| IBIS file generated by GenIBIS.exe Version 2.20
|   am37xxcbc
[IBIS ver]   4.1
[File name]   sprm510.ibs
[File Rev]   1.0
[Date]   Fri Jun 4, 2010, 5:00:00
[Source]   Data created at Texas Instruments
[Notes]   1) IBIS spec conformance checker (IBISCK4) ran with 0 errors
   and 576 warnings.  Warnings should be waived.
[Disclaimer] Please be aware that in the absence of a written agreement,
   Texas Instruments (TI) assumes no liability for: 1) the
   accuracy of the IBIS models provided to your company, 2) the
   proper functioning of these IBIS models in your design or for
   any resulting applications, or, 3) infringement of patents,
   copyrights, or intellectual property rights resulting from
   your use of these IBIS models. TI provides IBIS models as a
   service to our customers and therefore reserves the right to
   limit distribution of the IBIS models.
[Copyright]   Property of Texas Instruments Incorporated. Unauthorised
   reproduction and/or distribution is strictly prohibited. This
   product is protected under copyright law and trade secret law
   as an unpublished work. Created 1999,(C) Copyright 1999-2001,
   Texas Instruments Incorporated., All Rights Reserved. These
   commodities are under the U.S. Government distribution license
   control.As such,they are not to be re-exported without the
   prior approval of the U.S. Department of Commerce.
|   Component am37xxcbc
[Component]   am37xxcbc
[Manufacturer]   Texas Instruments.
[Package Model] am37xxcbc
[Package]
|   typ   min   max
R_pkg   0.66652835   4.09667e-02   1.29209e+00
L_pkg   4.458319E-009   -2.31662e-10   9.14830e-09
C_pkg   1.8121365E-012   -7.09787e-13   4.33406e-12
[Pin]   signal_name   model_name
D26   CAM_STROBE   Selector2
C25   CAM_XCLKA   Selector2
P25   CAM_D6   Selector11
N26   CAM_D9   Selector11
A24   CAM_D2   Selector16
P26   CAM_D7   Selector11
AE16   CAM_D0   Selector3
A23   CAM_WEN   Selector10
D23   CAM_VS   Selector10
C26   CAM_PCLK   Selector2
B24   CAM_D3   Selector16
B23   CAM_FLD   Selector10
AE15   CAM_D1   Selector3
E25   CAM_XCLKB   Selector2
D25   CAM_D10   Selector8
C24   CAM_D5   Selector16
C23   CAM_HS   Selector10
N25   CAM_D8   Selector11
E26   CAM_D11   Selector8
D24   CAM_D4   Selector16
AD17   gpio_112   Selector11
AD16   gpio_113   Selector11
AE17   gpio_115   Selector11
AE18   gpio_114   Selector11
M26   DSS_DATA19   Selector8
F26   DSS_ACBIAS   Selector8
AD26   DSS_DATA11   Selector16
AC25   DSS_DATA22   Selector16
L26   DSS_DATA17   Selector8
Y25   DSS_DATA13   Selector16
M25   DSS_VSYNC   Selector8
AE23   DSS_DATA2   Selector14
AC26   DSS_DATA10   Selector16
J26   DSS_DATA9   Selector8
AB26   DSS_DATA15   Selector16
K24   DSS_HSYNC   Selector8
AE21   DSS_DATA0   Selector13
AD24   DSS_DATA5   Selector14
AD23   DSS_DATA4   Selector14
M24   DSS_DATA18   Selector8
AA25   DSS_DATA12   Selector16
AE22   DSS_DATA1   Selector13
H25   DSS_DATA7   Selector8
AA26   DSS_DATA14   Selector16
G25   DSS_PCLK   Selector8
N24   DSS_DATA21   Selector8
L25   DSS_DATA16   Selector8
AB25   DSS_DATA23   Selector16
G26   DSS_DATA6   Selector8
AE24   DSS_DATA3   Selector14
F25   DSS_DATA20   Selector8
H26   DSS_DATA8   Selector8
AB3   ETK_CTL   Selector2
AD3   ETK_D2   Selector2
AE6   ETK_D12   Selector2
AF9   ETK_D14   Selector2
AE9   ETK_D15   Selector2
AE4   ETK_D10   Selector2
AF7   ETK_D13   Selector2
AC3   ETK_D0   Selector2
AB2   ETK_CLK   Selector2
Y3   ETK_D4   Selector2
V2   ETK_D9   Selector2
AD4   ETK_D1   Selector2
AA3   ETK_D3   Selector2
AD2   ETK_D7   Selector2
AA4   ETK_D8   Selector2
AF6   ETK_D11   Selector2
AE3   ETK_D6   Selector2
AB1   ETK_D5   Selector2
P1   GPMC_D13   Selector8
B6   GPMC_NCS3   Selector16
E2   GPMC_A8   Selector16
AD5   GPMC_D6   Selector8
B3   GPMC_WAIT2   Selector16
AC6   GPMC_NWP   Selector8
C4   GPMC_NCS5   Selector16
K2   GPMC_NBE0_CLE   Selector8
H2   GPMC_A3   Selector8
V1   GPMC_D8   Selector8
D1   GPMC_A9   Selector16
D2   GPMC_A10   Selector16
F2   GPMC_A6   Selector16
A4   GPMC_A11   Selector16
AC8   GPMC_WAIT1   Selector16
M2   GPMC_D15   Selector8
AD1   GPMC_NCS1   Selector16
AE5   GPMC_D4   Selector8
B5   GPMC_NCS6   Selector16
AA2   GPMC_D0   Selector8
AD6   GPMC_D5   Selector8
AD10   GPMC_NADV_ALE   Selector16
U2   GPMC_D11   Selector8
AA1   GPMC_D1   Selector8
B4   GPMC_NCS4   Selector16
C6   GPMC_WAIT3   Selector16
N2   GPMC_NOE   Selector16
AC5   GPMC_D7   Selector8
H1   GPMC_A2   Selector8
AC1   GPMC_D3   Selector8
Y1   GPMC_D9   Selector8
L2   GPMC_D14   Selector8
G2   GPMC_A4   Selector8
AD8   GPMC_NCS0   Selector16
E1   GPMC_A7   Selector16
AC11   GPMC_WAIT0   Selector16
M1   GPMC_NWE   Selector16
U1   GPMC_D12   Selector8
J1   GPMC_NBE1   Selector8
A3   GPMC_NCS2   Selector16
J2   GPMC_A1   Selector8
F1   GPMC_A5   Selector8
C5   GPMC_NCS7   Selector16
T1   GPMC_D10   Selector8
N1   GPMC_CLK   Selector8
AC2   GPMC_D2   Selector8
J23   HDQ_SIO   Selector5
W20   HSUSB0_DATA3   Selector2
V19   HSUSB0_DIR   Selector2
V20   HSUSB0_DATA0   Selector2
V18   HSUSB0_DATA2   Selector2
Y18   HSUSB0_DATA5   Selector2
U20   HSUSB0_STP   Selector2
W18   HSUSB0_NXT   Selector2
Y20   HSUSB0_DATA1   Selector2
W17   HSUSB0_DATA4   Selector2
Y17   HSUSB0_DATA7   Selector2
W19   HSUSB0_CLK   Selector19
Y19   HSUSB0_DATA6   Selector2
W16   I2C4_SDA   Selector20
AC4   I2C3_SDA   Selector17
C2   I2C2_SCL   Selector17
AD15   I2C4_SCL   Selector20
J24   I2C1_SDA   Selector17
C1   I2C2_SDA   Selector17
J25   I2C1_SCL   Selector17
AB4   I2C3_SCL   Selector17
Y15   JTAG_EMU0   Selector1
U16   JTAG_TDI   Selector1
U15   JTAG_NTRST   Selector1
V14   JTAG_TCK   Selector1
V15   JTAG_TMS_TMSC   Selector1
Y13   JTAG_TDO   Selector1
W13   JTAG_RTCK   Selector1
Y14   JTAG_EMU1   Selector1
T19   MCBSP_CLKS   Selector2
V17   MCBSP1_FSR   Selector2
P20   MCBSP1_FSX   Selector2
T17   MCBSP1_CLKX   Selector2
U19   MCBSP1_CLKR   Selector2
U17   MCBSP1_DX   Selector2
T20   MCBSP1_DR   Selector2
R18   MCBSP2_CLKX   Selector2
U18   MCBSP2_FSX   Selector2
T18   MCBSP2_DR   Selector2
R19   MCBSP2_DX   Selector2
W3   MCBSP3_FSX   Selector2
U3   MCBSP3_CLKX   Selector2
P3   MCBSP3_DX   Selector2
N3   MCBSP3_DR   Selector2
U4   MCBSP4_DR   Selector2
V3   MCBSP4_CLKX   Selector2
R3   MCBSP4_DX   Selector2
T3   MCBSP4_FSX   Selector2
R9   MCSPI1_CS2   Selector2
T8   MCSPI1_CS3   Selector2
P8   MCSPI1_SIMO   Selector2
R8   MCSPI1_CS1   Selector2
P7   MCSPI1_SOMI   Selector2
P9   MCSPI1_CLK   Selector2
R7   MCSPI1_CS0   Selector2
W7   MCSPI2_CLK   Selector2
V9   MCSPI2_CS1   Selector2
V8   MCSPI2_CS0   Selector2
U8   MCSPI2_SOMI   Selector2
W8   MCSPI2_SIMO   Selector2
L18   MMC1_CMD   Selector15
K18   MMC1_DAT2   Selector15
N19   MMC1_CLK   Selector15
M19   MMC1_DAT0   Selector15
M18   MMC1_DAT1   Selector15
N20   MMC1_DAT3   Selector15
V10   MMC2_DAT4   Selector2
T9   MMC2_DAT1   Selector2
R10   MMC2_CMD   Selector2
T10   MMC2_DAT0   Selector2
L3   MMC2_DAT6   Selector2
U9   MMC2_DAT3   Selector2
W10   MMC2_CLK   Selector2
U10   MMC2_DAT2   Selector2
K3   MMC2_DAT7   Selector2
M3   MMC2_DAT5   Selector2
P18   gpio_128   Selector4
P19   gpio_129   Selector6
M20   gpio_126   Selector6
P17   gpio_127   Selector6
W15   SYS_CLKREQ   Selector7
E3   SYS_BOOT3   Selector8
D3   SYS_BOOT1   Selector8
G3   SYS_BOOT5   Selector8
AE20   SYS_32K   Selector7
V16   SYS_NIRQ   Selector18
V13   SYS_NRESPWRON   Model225
AD7   SYS_NRESWARM   Selector9
AF19   SYS_XTALIN   Model1
AE14   SYS_CLKOUT1   Selector12
C3   SYS_BOOT2   Selector8
D4   SYS_BOOT6   Selector16
E4   SYS_BOOT4   Selector8
F3   SYS_BOOT0   Selector8
V12   SYS_OFF_MODE   Selector12
W11   SYS_CLKOUT2   Selector10
R2   UART1_RTS   Selector2
H3   UART1_RX   Selector2
L4   UART1_TX   Selector2
W2   UART1_CTS   Selector2
AA24   UART2_RTS   Selector10
Y24   UART2_CTS   Selector10
AD22   UART2_TX   Selector10
AD21   UART2_RX   Selector10
H24   UART3_RX_IRRX   Selector5
G24   UART3_TX_IRTX   Selector21
F23   UART3_CTS_RCTX   Selector5
F24   UART3_RTS_SD   Selector21
| Device pads which are not required to be modeled. Included for completeness
|A18   POWER
|AB24   POWER
|AC15   POWER
|AC18   POWER
|AC24   POWER
|AC7   POWER
|AD18   POWER
|AD19   POWER
|AD20   POWER
|AE10   POWER
|C11   POWER
|D9   POWER
|E24   POWER
|G4   POWER
|J15   POWER
|J18   POWER
|L20   POWER
|L24   POWER
|L7   POWER
|M4   POWER
|T24   POWER
|T4   POWER
|W24   POWER
|Y4   POWER
|AE19   CAP_VDDU_ARRAY   POWER
|K20   CAP_VDD_SRAM_CORE   POWER
|N9   CAP_VDD_SRAM_MPU_IVA POWER
|K14   CAP_VDD_WKUP_LOGIC   POWER
|D6   CAP_VDD_BB_MPU_IVA   POWER
|AF23   SYS_XTALGND   KELVINGROUND
|AC21   VDD_CORE   POWER
|D15   VDD_CORE   POWER
|G11   VDD_CORE   POWER
|G18   VDD_CORE   POWER
|H20   VDD_CORE   POWER
|M17   VDD_CORE   POWER
|M7   VDD_CORE   POWER
|R20   VDD_CORE   POWER
|T7   VDD_CORE   POWER
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[Model Selector] Selector1
Model2 1.8V-I/O-PD-X-1.8V +5/-10%
Model3 1.8V-I/O-PI-X-1.8V +5/-10%V
Model4 1.8V-I/O-PU-X-1.8V +5/-10%
|   Usage I#1.8V#PD/PI/PU#LB0/LB1#BQ1850OMAPSMART2HYFBPB_SSBHH
[Model Selector] Selector2
Model10 1.8V-I/O-PI-LB1-1.8 +5/-10%
Model5 1.8V-I/O-PI-LB0-1.8 +5/-10%
Model6 1.8V-I/O-PU-LB0-1.8 +5/-10%
Model7 1.8V-I/O-PD-LB0-1.8 +5/-10%
Model8 1.8V-I/O-PU-LB1-1.8 +5/-10%
Model9 1.8V-I/O-PD-LB1-1.8 +5/-10%
|   Usage I#1.8V#PD/PI/PU##CAMERARX_ADDON.DY3
[Model Selector] Selector3
Model11 1.8V-INPUT-PD-X-1.8V +5/-10%
Model12 1.8V-INPUT-PI-X-1.8V +5/-10%
Model13 1.8V-INPUT-PU-X-1.8V +5/-10%
|   Usage O#1.8V#PD/PI/PU#SC00LB00/SC00LB01/SC01LB10/SC01LB11/SC10LB10/SC10LB11#BQ18OMAPSMART1HYFBPBNOPM_SSBHH
[Model Selector] Selector4
Model14 1.8V-I/O-PI-SC00LB00-1.8 +5/-10%
Model15 1.8V-I/O-PU-SC00LB00-1.8 +5/-10%
Model16 1.8V-I/O-PD-SC00LB00-1.8 +5/-10%
Model17 1.8V-I/O-PU-SC00LB01-1.8 +5/-10%
Model18 1.8V-I/O-PD-SC00LB01-1.8 +5/-10%
Model19 1.8V-I/O-PI-SC00LB01-1.8 +5/-10%
Model20 1.8V-I/O-PD-SC01LB10-1.8 +5/-10%
Model21 1.8V-I/O-PI-SC01LB10-1.8 +5/-10%
Model22 1.8V-I/O-PU-SC01LB10-1.8 +5/-10%
Model23 1.8V-I/O-PD-SC01LB11-1.8 +5/-10%
Model24 1.8V-I/O-PU-SC01LB11-1.8 +5/-10%
Model25 1.8V-I/O-PI-SC01LB11-1.8 +5/-10%
Model26 1.8V-I/O-PI-SC10LB10-1.8 +5/-10%
Model27 1.8V-I/O-PU-SC10LB10-1.8 +5/-10%
Model28 1.8V-I/O-PD-SC10LB10-1.8 +5/-10%
Model29 1.8V-I/O-PU-SC10LB11-1.8 +5/-10%
Model30 1.8V-I/O-PI-SC10LB11-1.8 +5/-10%
Model31 1.8V-I/O-PD-SC10LB11-1.8 +5/-10%
|   Usage I#1.8V#PD/PI/PU#SC00LB00/SC00LB01/SC01LB10/SC01LB11/SC10LB10/SC10LB11#BQ18OMAPSMART1HYFBPB_SSBHH
[Model Selector] Selector5
Model32 1.8V-I/O-PD-SC01LB11-1.8 +5/-10%
Model33 1.8V-I/O-PD-SC01LB10-1.8 +5/-10%
Model34 1.8V-I/O-PD-SC00LB11-1.8 +5/-10%
Model35 1.8V-I/O-PD-SC00LB10-1.8 +5/-10%
Model36 1.8V-I/O-PD-SC00LB01-1.8 +5/-10%
Model37 1.8V-I/O-PD-SC10LB01-1.8 +5/-10%
Model38 1.8V-I/O-PD-SC10LB00-1.8 +5/-10%
Model39 1.8V-I/O-PD-SC01LB01-1.8 +5/-10%
Model40 1.8V-I/O-PD-SC01LB00-1.8 +5/-10%
Model41 1.8V-I/O-PD-SC00LB00-1.8 +5/-10%
Model42 1.8V-I/O-PD-SC10LB11-1.8 +5/-10%
Model43 1.8V-I/O-PD-SC10LB10-1.8 +5/-10%
Model44 1.8V-I/O-PI-SC10LB10-1.8 +5/-10%
Model45 1.8V-I/O-PI-SC10LB01-1.8 +5/-10%
Model46 1.8V-I/O-PI-SC10LB00-1.8 +5/-10%
Model47 1.8V-I/O-PI-SC01LB10-1.8 +5/-10%
Model48 1.8V-I/O-PI-SC01LB01-1.8 +5/-10%
Model49 1.8V-I/O-PI-SC01LB00-1.8 +5/-10%
Model50 1.8V-I/O-PI-SC00LB01-1.8 +5/-10%
Model51 1.8V-I/O-PI-SC00LB00-1.8 +5/-10%
Model52 1.8V-I/O-PI-SC10LB11-1.8 +5/-10%
Model53 1.8V-I/O-PI-SC01LB11-1.8 +5/-10%
Model54 1.8V-I/O-PI-SC00LB11-1.8 +5/-10%
Model55 1.8V-I/O-PI-SC00LB10-1.8 +5/-10%
Model56 1.8V-I/O-PU-SC00LB01-1.8 +5/-10%
Model57 1.8V-I/O-PU-SC10LB11-1.8 +5/-10%
Model58 1.8V-I/O-PU-SC10LB10-1.8 +5/-10%
Model59 1.8V-I/O-PU-SC01LB11-1.8 +5/-10%
Model60 1.8V-I/O-PU-SC01LB10-1.8 +5/-10%
Model61 1.8V-I/O-PU-SC00LB00-1.8 +5/-10%
Model62 1.8V-I/O-PU-SC10LB01-1.8 +5/-10%
Model63 1.8V-I/O-PU-SC10LB00-1.8 +5/-10%
Model64 1.8V-I/O-PU-SC00LB11-1.8 +5/-10%
Model65 1.8V-I/O-PU-SC01LB01-1.8 +5/-10%
Model66 1.8V-I/O-PU-SC00LB10-1.8 +5/-10%
Model67 1.8V-I/O-PU-SC01LB00-1.8 +5/-10%
|   Usage IO#1.8V/3V#PD/PI/PU##BQUSIM1833DVHYPBFZLP18NOPM_SSCHH
[Model Selector] Selector6
Model68 1.8V-I/O-PD-X-+5/-10%V
Model69 1.8V-I/O-PU-X-+5/-10%V
Model70 1.8V-I/O-PI-X-+5/-10%V
Model71 3V-I/O-PD-X-3V+-10%
Model72 3V-I/O-PU-X-3V+-10%
Model73 3V-I/O-PI-X-3V+-10%
|   Usage I#1.8V#PD/PI/PU#SC00LB00/SC00LB01/SC01LB10/SC01LB11/SC10LB10/SC10LB11#BQ18OMAPSMART1HYFBPBNOPM_SSBHV
[Model Selector] Selector7
Model100 1.8V-I/O-PU-SC10LB10-1.8 +5/-10%
Model101 1.8V-I/O-PU-SC01LB11-1.8 +5/-10%
Model102 1.8V-I/O-PU-SC01LB10-1.8 +5/-10%
Model103 1.8V-I/O-PU-SC00LB00-1.8 +5/-10%
Model104 1.8V-I/O-PU-SC10LB01-1.8 +5/-10%
Model105 1.8V-I/O-PU-SC10LB00-1.8 +5/-10%
Model106 1.8V-I/O-PU-SC00LB11-1.8 +5/-10%
Model107 1.8V-I/O-PU-SC01LB01-1.8 +5/-10%
Model108 1.8V-I/O-PU-SC00LB10-1.8 +5/-10%
Model109 1.8V-I/O-PU-SC01LB00-1.8 +5/-10%
Model74 1.8V-I/O-PD-SC01LB11-1.8 +5/-10%
Model75 1.8V-I/O-PD-SC01LB10-1.8 +5/-10%
Model76 1.8V-I/O-PD-SC00LB11-1.8 +5/-10%
Model77 1.8V-I/O-PD-SC00LB10-1.8 +5/-10%
Model78 1.8V-I/O-PD-SC00LB01-1.8 +5/-10%
Model79 1.8V-I/O-PD-SC10LB01-1.8 +5/-10%
Model80 1.8V-I/O-PD-SC10LB00-1.8 +5/-10%
Model81 1.8V-I/O-PD-SC01LB01-1.8 +5/-10%
Model82 1.8V-I/O-PD-SC01LB00-1.8 +5/-10%
Model83 1.8V-I/O-PD-SC00LB00-1.8 +5/-10%
Model84 1.8V-I/O-PD-SC10LB11-1.8 +5/-10%
Model85 1.8V-I/O-PD-SC10LB10-1.8 +5/-10%
Model86 1.8V-I/O-PI-SC10LB10-1.8 +5/-10%
Model87 1.8V-I/O-PI-SC10LB01-1.8 +5/-10%
Model88 1.8V-I/O-PI-SC10LB00-1.8 +5/-10%
Model89 1.8V-I/O-PI-SC01LB10-1.8 +5/-10%
Model90 1.8V-I/O-PI-SC01LB01-1.8 +5/-10%
Model91 1.8V-I/O-PI-SC01LB00-1.8 +5/-10%
Model92 1.8V-I/O-PI-SC00LB01-1.8 +5/-10%
Model93 1.8V-I/O-PI-SC00LB00-1.8 +5/-10%
Model94 1.8V-I/O-PI-SC10LB11-1.8 +5/-10%
Model95 1.8V-I/O-PI-SC01LB11-1.8 +5/-10%
Model96 1.8V-I/O-PI-SC00LB11-1.8 +5/-10%
Model97 1.8V-I/O-PI-SC00LB10-1.8 +5/-10%
Model98 1.8V-I/O-PU-SC00LB01-1.8 +5/-10%
Model99 1.8V-I/O-PU-SC10LB11-1.8 +5/-10%
|   Usage O#1.8V#PD/PI/PU#LB0/LB1#BQ18OMAPSMART2HYFBPB_SSBHH
[Model Selector] Selector8
Model110 1.8V-I/O-PD-LB1-1.8 +5/-10%
Model111 1.8V-I/O-PD-LB0-1.8 +5/-10%
Model112 1.8V-I/O-PI-LB0-1.8 +5/-10%
Model113 1.8V-I/O-PI-LB1-1.8 +5/-10%
Model114 1.8V-I/O-PU-LB1-1.8 +5/-10%
Model115 1.8V-I/O-PU-LB0-1.8 +5/-10%
|   Usage IO#1.8V#PD/PI/PU##BQOMAPGFR50CHYFBPBNOPM_SSBHV
[Model Selector] Selector9
Model116 1.8V-I/O-PD-X-+5/-10%V
Model117 1.8V-I/O-PI-X-+5/-10%V
Model118 1.8V-I/O-PU-X-+5/-10%V
|   Usage IO#1.8V#PD/PI/PU#LB0/LB1#BQ1850OMAPSMART2HYFBPB_SSBHV
[Model Selector] Selector10
Model119 1.8V-I/O-PI-LB0-1.8 +5/-10%
Model120 1.8V-I/O-PU-LB0-1.8 +5/-10%
Model121 1.8V-I/O-PD-LB0-1.8 +5/-10%
Model122 1.8V-I/O-PU-LB1-1.8 +5/-10%
Model123 1.8V-I/O-PD-LB1-1.8 +5/-10%
Model124 1.8V-I/O-PI-LB1-1.8 +5/-10%
|   Usage I#1.8V#PD/PI/PU##CAMERARX_CORE.YAGPI
[Model Selector] Selector11
Model125 1.8V-INPUT-PD-X-1.8V +5/-10%
Model126 1.8V-INPUT-PI-X-1.8V +5/-10%
Model127 1.8V-INPUT-PU-X-1.8V +5/-10%
|   Usage O#1.8V#PD/PI/PU#SC00LB00/SC00LB01/SC01LB10/SC01LB11/SC10LB10/SC10LB11#BQ18OMAPSMART1HYFBPBNOPM_SSBHV
[Model Selector] Selector12
Model100 1.8V-I/O-PU-SC10LB10-1.8 +5/-10%
Model101 1.8V-I/O-PU-SC01LB11-1.8 +5/-10%
Model102 1.8V-I/O-PU-SC01LB10-1.8 +5/-10%
Model103 1.8V-I/O-PU-SC00LB00-1.8 +5/-10%
Model74 1.8V-I/O-PD-SC01LB11-1.8 +5/-10%
Model75 1.8V-I/O-PD-SC01LB10-1.8 +5/-10%
Model78 1.8V-I/O-PD-SC00LB01-1.8 +5/-10%
Model83 1.8V-I/O-PD-SC00LB00-1.8 +5/-10%
Model84 1.8V-I/O-PD-SC10LB11-1.8 +5/-10%
Model85 1.8V-I/O-PD-SC10LB10-1.8 +5/-10%
Model86 1.8V-I/O-PI-SC10LB10-1.8 +5/-10%
Model89 1.8V-I/O-PI-SC01LB10-1.8 +5/-10%
Model92 1.8V-I/O-PI-SC00LB01-1.8 +5/-10%
Model93 1.8V-I/O-PI-SC00LB00-1.8 +5/-10%
Model94 1.8V-I/O-PI-SC10LB11-1.8 +5/-10%
Model95 1.8V-I/O-PI-SC01LB11-1.8 +5/-10%
Model98 1.8V-I/O-PU-SC00LB01-1.8 +5/-10%
Model99 1.8V-I/O-PU-SC10LB11-1.8 +5/-10%
|   Usage IO#1.8V#PD/PI/PU#SC00LB00/SC00LB01/SC01LB10/SC01LB11/SC10LB10/SC10LB11#DSIPHY_WIO_ADDON_GPIOWRAPPER.GPI
[Model Selector] Selector13
Model128 1.8V-I/O-PD-SC01LB11-1.8 +5/-10%
Model129 1.8V-I/O-PD-SC01LB10-1.8 +5/-10%
Model130 1.8V-I/O-PD-SC00LB11-1.8 +5/-10%
Model131 1.8V-I/O-PD-SC00LB10-1.8 +5/-10%
Model132 1.8V-I/O-PD-SC00LB01-1.8 +5/-10%
Model133 1.8V-I/O-PD-SC10LB01-1.8 +5/-10%
Model134 1.8V-I/O-PD-SC10LB00-1.8 +5/-10%
Model135 1.8V-I/O-PD-SC01LB01-1.8 +5/-10%
Model136 1.8V-I/O-PD-SC01LB00-1.8 +5/-10%
Model137 1.8V-I/O-PD-SC00LB00-1.8 +5/-10%
Model138 1.8V-I/O-PD-SC10LB11-1.8 +5/-10%
Model139 1.8V-I/O-PD-SC10LB10-1.8 +5/-10%
Model140 1.8V-I/O-PI-SC10LB10-1.8 +5/-10%
Model141 1.8V-I/O-PI-SC10LB01-1.8 +5/-10%
Model142 1.8V-I/O-PI-SC10LB00-1.8 +5/-10%
Model143 1.8V-I/O-PI-SC01LB10-1.8 +5/-10%
Model144 1.8V-I/O-PI-SC01LB01-1.8 +5/-10%
Model145 1.8V-I/O-PI-SC01LB00-1.8 +5/-10%
Model146 1.8V-I/O-PI-SC00LB01-1.8 +5/-10%
Model147 1.8V-I/O-PI-SC00LB00-1.8 +5/-10%
Model148 1.8V-I/O-PI-SC10LB11-1.8 +5/-10%
Model149 1.8V-I/O-PI-SC01LB11-1.8 +5/-10%
Model150 1.8V-I/O-PI-SC00LB11-1.8 +5/-10%
Model151 1.8V-I/O-PI-SC00LB10-1.8 +5/-10%
Model152 1.8V-I/O-PU-SC00LB01-1.8 +5/-10%
Model153 1.8V-I/O-PU-SC10LB11-1.8 +5/-10%
Model154 1.8V-I/O-PU-SC10LB10-1.8 +5/-10%
Model155 1.8V-I/O-PU-SC01LB11-1.8 +5/-10%
Model156 1.8V-I/O-PU-SC01LB10-1.8 +5/-10%
Model157 1.8V-I/O-PU-SC00LB00-1.8 +5/-10%
Model158 1.8V-I/O-PU-SC10LB01-1.8 +5/-10%
Model159 1.8V-I/O-PU-SC10LB00-1.8 +5/-10%
Model160 1.8V-I/O-PU-SC00LB11-1.8 +5/-10%
Model161 1.8V-I/O-PU-SC01LB01-1.8 +5/-10%
Model162 1.8V-I/O-PU-SC00LB10-1.8 +5/-10%
Model163 1.8V-I/O-PU-SC01LB00-1.8 +5/-10%
|   Usage IO#1.8V#PD/PI/PU#SC00LB00/SC00LB01/SC01LB10/SC01LB11/SC10LB10/SC10LB11#DSIPHY_WIO_CORE_GPIOWRAPPER.GPI
[Model Selector] Selector14
Model176 1.8V-I/O-PD-SC01LB11-1.8 +5/-10%
Model177 1.8V-I/O-PD-SC01LB10-1.8 +5/-10%
Model178 1.8V-I/O-PD-SC00LB11-1.8 +5/-10%
Model179 1.8V-I/O-PD-SC00LB10-1.8 +5/-10%
Model180 1.8V-I/O-PD-SC00LB01-1.8 +5/-10%
Model181 1.8V-I/O-PD-SC10LB01-1.8 +5/-10%
Model182 1.8V-I/O-PD-SC10LB00-1.8 +5/-10%
Model183 1.8V-I/O-PD-SC01LB01-1.8 +5/-10%
Model184 1.8V-I/O-PD-SC01LB00-1.8 +5/-10%
Model185 1.8V-I/O-PD-SC00LB00-1.8 +5/-10%
Model186 1.8V-I/O-PD-SC10LB11-1.8 +5/-10%
Model187 1.8V-I/O-PD-SC10LB10-1.8 +5/-10%
Model188 1.8V-I/O-PI-SC10LB10-1.8 +5/-10%
Model189 1.8V-I/O-PI-SC10LB01-1.8 +5/-10%
Model190 1.8V-I/O-PI-SC10LB00-1.8 +5/-10%
Model191 1.8V-I/O-PI-SC01LB10-1.8 +5/-10%
Model192 1.8V-I/O-PI-SC01LB01-1.8 +5/-10%
Model193 1.8V-I/O-PI-SC01LB00-1.8 +5/-10%
Model194 1.8V-I/O-PI-SC00LB01-1.8 +5/-10%
Model195 1.8V-I/O-PI-SC00LB00-1.8 +5/-10%
Model196 1.8V-I/O-PI-SC10LB11-1.8 +5/-10%
Model197 1.8V-I/O-PI-SC01LB11-1.8 +5/-10%
Model198 1.8V-I/O-PI-SC00LB11-1.8 +5/-10%
Model199 1.8V-I/O-PI-SC00LB10-1.8 +5/-10%
Model200 1.8V-I/O-PU-SC00LB01-1.8 +5/-10%
Model201 1.8V-I/O-PU-SC10LB11-1.8 +5/-10%
Model202 1.8V-I/O-PU-SC10LB10-1.8 +5/-10%
Model203 1.8V-I/O-PU-SC01LB11-1.8 +5/-10%
Model204 1.8V-I/O-PU-SC01LB10-1.8 +5/-10%
Model205 1.8V-I/O-PU-SC00LB00-1.8 +5/-10%
Model206 1.8V-I/O-PU-SC10LB01-1.8 +5/-10%
Model207 1.8V-I/O-PU-SC10LB00-1.8 +5/-10%
Model208 1.8V-I/O-PU-SC00LB11-1.8 +5/-10%
Model209 1.8V-I/O-PU-SC01LB01-1.8 +5/-10%
Model210 1.8V-I/O-PU-SC00LB10-1.8 +5/-10%
Model211 1.8V-I/O-PU-SC01LB00-1.8 +5/-10%
|   Usage O#1.8V/3V#PD/PI/PU#SC0/SC1#BQMMC1833DVHYPBFZLP18_SSCHH
[Model Selector] Selector15
Model164 1.8V-I/O-PD-SC0-1.8V +5/-10%
Model165 1.8V-I/O-PD-SC1-1.8V +5/-10%
Model166 1.8V-I/O-PI-SC0-1.8V +5/-10%
Model167 1.8V-I/O-PI-SC1-1.8V +5/-10%
Model168 1.8V-I/O-PU-SC0-1.8V +5/-10%
Model169 1.8V-I/O-PU-SC1-1.8V +5/-10%
Model170 3V-I/O-PD-SC0-3V +-10%
Model171 3V-I/O-PD-SC1-3V +-10%
Model172 3V-I/O-PI-SC0-3V +-10%
Model173 3V-I/O-PI-SC1-3V +-10%
Model174 3V-I/O-PU-SC0-3V +-10%
Model175 3V-I/O-PU-SC1-3V +-10%
|   Usage I#1.8V#PD/PI/PU#LB0/LB1#BQ18OMAPSMART2HYFBPB_SSBHV
[Model Selector] Selector16
Model212 1.8V-I/O-PD-LB1-1.8 +5/-10%
Model213 1.8V-I/O-PD-LB0-1.8 +5/-10%
Model214 1.8V-I/O-PI-LB0-1.8 +5/-10%
Model215 1.8V-I/O-PI-LB1-1.8 +5/-10%
Model216 1.8V-I/O-PU-LB1-1.8 +5/-10%
Model217 1.8V-I/O-PU-LB0-1.8 +5/-10%
|   Usage IO#1.8V#PI/PU#LB00/LB01/LB10#BQOMAPI2CHYFBPBRES_SSBHH
[Model Selector] Selector17
Model218 1.8V-I/O_OPEN_DRAIN-PI-LB00-1.8V +5/-10%
Model219 1.8V-I/O_OPEN_DRAIN-PI-LB00-1.8V +5/-10%
Model220 1.8V-I/O-PU-LB00-1.8V +5/-10%
Model221 1.8V-I/O_OPEN_DRAIN-PU-LB01-1.8V +5/-10%
Model222 1.8V-I/O_OPEN_DRAIN-PU-LB10-1.8V +5/-10%
Model223 1.8V-I/O_OPEN_DRAIN-PU-LB00-1.8V +5/-10%
Model224 1.8V-I/O_OPEN_DRAIN-PU-LB00-1.8V +5/-10%
|   Usage I#1.8V#PD/PI/PU#SC00LB00/SC00LB01/SC01LB10/SC01LB11/SC10LB10/SC10LB11#BQ18OMAPSMART1HYFBPB_SSBHV
[Model Selector] Selector18
Model232 1.8V-I/O-PD-SC01LB11-1.8 +5/-10%
Model233 1.8V-I/O-PD-SC01LB10-1.8 +5/-10%
Model234 1.8V-I/O-PD-SC00LB11-1.8 +5/-10%
Model235 1.8V-I/O-PD-SC00LB01-1.8 +5/-10%
Model236 1.8V-I/O-PD-SC10LB01-1.8 +5/-10%
Model237 1.8V-I/O-PD-SC10LB00-1.8 +5/-10%
Model238 1.8V-I/O-PD-SC01LB01-1.8 +5/-10%
Model239 1.8V-I/O-PD-SC00LB00-1.8 +5/-10%
Model240 1.8V-I/O-PD-SC10LB11-1.8 +5/-10%
Model241 1.8V-I/O-PD-SC10LB10-1.8 +5/-10%
Model242 1.8V-I/O-PI-SC10LB10-1.8 +5/-10%
Model243 1.8V-I/O-PI-SC10LB01-1.8 +5/-10%
Model244 1.8V-I/O-PI-SC10LB00-1.8 +5/-10%
Model245 1.8V-I/O-PI-SC01LB10-1.8 +5/-10%
Model246 1.8V-I/O-PI-SC01LB01-1.8 +5/-10%
Model247 1.8V-I/O-PI-SC00LB01-1.8 +5/-10%
Model248 1.8V-I/O-PI-SC00LB00-1.8 +5/-10%
Model249 1.8V-I/O-PI-SC10LB11-1.8 +5/-10%
Model250 1.8V-I/O-PI-SC01LB11-1.8 +5/-10%
Model251 1.8V-I/O-PI-SC00LB11-1.8 +5/-10%
Model252 1.8V-I/O-PI-SC00LB10-1.8 +5/-10%
Model253 1.8V-I/O-PU-SC00LB01-1.8 +5/-10%
Model254 1.8V-I/O-PU-SC10LB11-1.8 +5/-10%
Model255 1.8V-I/O-PU-SC10LB10-1.8 +5/-10%
Model256 1.8V-I/O-PU-SC01LB11-1.8 +5/-10%
Model257 1.8V-I/O-PU-SC01LB10-1.8 +5/-10%
Model258 1.8V-I/O-PU-SC00LB00-1.8 +5/-10%
Model259 1.8V-I/O-PU-SC10LB01-1.8 +5/-10%
Model260 1.8V-I/O-PU-SC10LB00-1.8 +5/-10%
Model261 1.8V-I/O-PU-SC00LB11-1.8 +5/-10%
Model262 1.8V-I/O-PU-SC01LB01-1.8 +5/-10%
Model263 1.8V-I/O-PU-SC00LB10-1.8 +5/-10%
Model264 1.8V-I/O-PU-SC01LB00-1.8 +5/-10%
|   Usage I#1.8V#PD/PI/PU#LB0/LB1#BQ18OMAPSMART2FBPB_SSBHH
[Model Selector] Selector19
Model226 1.8V-I/O-PD-LB1-1.8 +5/-10%
Model227 1.8V-I/O-PD-LB0-1.8 +5/-10%
Model228 1.8V-I/O-PI-LB0-1.8 +5/-10%
Model229 1.8V-I/O-PI-LB1-1.8 +5/-10%
Model230 1.8V-I/O-PU-LB1-1.8 +5/-10%
Model231 1.8V-I/O-PU-LB0-1.8 +5/-10%
|   Usage IO#1.8V#PI/PU#LB00/LB01/LB10#BQOMAPI2CHYFBPBRESNOPM_SSBHV
[Model Selector] Selector20
Model265 1.8V-I/O_OPEN_DRAIN-PI-LB00-1.8V +5/-10%
Model266 1.8V-I/O_OPEN_DRAIN-PI-LB00-1.8V +5/-10%
Model267 1.8V-I/O-PU-LB00-1.8V +5/-10%
Model268 1.8V-I/O_OPEN_DRAIN-PU-LB01-1.8V +5/-10%
Model269 1.8V-I/O_OPEN_DRAIN-PU-LB10-1.8V +5/-10%
Model270 1.8V-I/O_OPEN_DRAIN-PU-LB00-1.8V +5/-10%
Model271 1.8V-I/O_OPEN_DRAIN-PU-LB00-1.8V +5/-10%
|   Usage O#1.8V#PD/PI/PU#SC00LB00/SC00LB01/SC01LB10/SC01LB11/SC10LB10/SC10LB11#BQ18OMAPSMART1HYFBPB_SSBHH
[Model Selector] Selector21
Model32 1.8V-I/O-PD-SC01LB11-1.8 +5/-10%
Model33 1.8V-I/O-PD-SC01LB10-1.8 +5/-10%
Model36 1.8V-I/O-PD-SC00LB01-1.8 +5/-10%
Model41 1.8V-I/O-PD-SC00LB00-1.8 +5/-10%
Model42 1.8V-I/O-PD-SC10LB11-1.8 +5/-10%
Model43 1.8V-I/O-PD-SC10LB10-1.8 +5/-10%
Model44 1.8V-I/O-PI-SC10LB10-1.8 +5/-10%
Model47 1.8V-I/O-PI-SC01LB10-1.8 +5/-10%
Model50 1.8V-I/O-PI-SC00LB01-1.8 +5/-10%
Model51 1.8V-I/O-PI-SC00LB00-1.8 +5/-10%
Model52 1.8V-I/O-PI-SC10LB11-1.8 +5/-10%
Model53 1.8V-I/O-PI-SC01LB11-1.8 +5/-10%
Model56 1.8V-I/O-PU-SC00LB01-1.8 +5/-10%
Model57 1.8V-I/O-PU-SC10LB11-1.8 +5/-10%
Model58 1.8V-I/O-PU-SC10LB10-1.8 +5/-10%
Model59 1.8V-I/O-PU-SC01LB11-1.8 +5/-10%
Model60 1.8V-I/O-PU-SC01LB10-1.8 +5/-10%
Model61 1.8V-I/O-PU-SC00LB00-1.8 +5/-10%
| Package model definition
[Define Package Model]  am37xxcbc
[Manufacturer]   Texas Instruments.
[OEM]   Texas Instruments.
[Description]   am37xxcbc package model generated by GenIBIS.exe
[Number Of Pins]   224
[Pin Numbers]
D26   | 1 CAM_STROBE   O
C25   | 2 CAM_XCLKA   O
P25   | 3 CAM_D6   I
N26   | 4 CAM_D9   I
A24   | 5 CAM_D2   I
P26   | 6 CAM_D7   I
AE16   | 7 CAM_D0   I
A23   | 8 CAM_WEN   I
D23   | 9 CAM_VS   IO
C26   | 10 CAM_PCLK   I
B24   | 11 CAM_D3   I
B23   | 12 CAM_FLD   IO
AE15   | 13 CAM_D1   I
E25   | 14 CAM_XCLKB   O
D25   | 15 CAM_D10   I
C24   | 16 CAM_D5   I
C23   | 17 CAM_HS   IO
N25   | 18 CAM_D8   I
E26   | 19 CAM_D11   I
D24   | 20 CAM_D4   I
AD17   | 21 gpio_112   I
AD16   | 22 gpio_113   I
AE17   | 23 gpio_115   I
AE18   | 24 gpio_114   I
M26   | 25 DSS_DATA19   IO
F26   | 26 DSS_ACBIAS   O
AD26   | 27 DSS_DATA11   IO
AC25   | 28 DSS_DATA22   O
L26   | 29 DSS_DATA17   IO
Y25   | 30 DSS_DATA13   IO
M25   | 31 DSS_VSYNC   O
AE23   | 32 DSS_DATA2   IO
AC26   | 33 DSS_DATA10   IO
J26   | 34 DSS_DATA9   IO
AB26   | 35 DSS_DATA15   IO
K24   | 36 DSS_HSYNC   O
AE21   | 37 DSS_DATA0   IO
AD24   | 38 DSS_DATA5   IO
AD23   | 39 DSS_DATA4   IO
M24   | 40 DSS_DATA18   IO
AA25   | 41 DSS_DATA12   IO
AE22   | 42 DSS_DATA1   IO
H25   | 43 DSS_DATA7   IO
AA26   | 44 DSS_DATA14   IO
G25   | 45 DSS_PCLK   O
N24   | 46 DSS_DATA21   O
L25   | 47 DSS_DATA16   IO
AB25   | 48 DSS_DATA23   O
G26   | 49 DSS_DATA6   IO
AE24   | 50 DSS_DATA3   IO
F25   | 51 DSS_DATA20   O
H26   | 52 DSS_DATA8   IO
AB3   | 53 ETK_CTL   O
AD3   | 54 ETK_D2   O
AE6   | 55 ETK_D12   O
AF9   | 56 ETK_D14   O
AE9   | 57 ETK_D15   O
AE4   | 58 ETK_D10   O
AF7   | 59 ETK_D13   O
AC3   | 60 ETK_D0   O
AB2   | 61 ETK_CLK   O
Y3   | 62 ETK_D4   O
V2   | 63 ETK_D9   O
AD4   | 64 ETK_D1   O
AA3   | 65 ETK_D3   O
AD2   | 66 ETK_D7   O
AA4   | 67 ETK_D8   O
AF6   | 68 ETK_D11   O
AE3   | 69 ETK_D6   O
AB1   | 70 ETK_D5   O
P1   | 71 GPMC_D13   IO
B6   | 72 GPMC_NCS3   O
E2   | 73 GPMC_A8   O
AD5   | 74 GPMC_D6   IO
B3   | 75 GPMC_WAIT2   I
AC6   | 76 GPMC_NWP   O
C4   | 77 GPMC_NCS5   O
K2   | 78 GPMC_NBE0_CLE   O
H2   | 79 GPMC_A3   O
V1   | 80 GPMC_D8   IO
D1   | 81 GPMC_A9   O
D2   | 82 GPMC_A10   O
F2   | 83 GPMC_A6   O
A4   | 84 GPMC_A11   IO
AC8   | 85 GPMC_WAIT1   I
M2   | 86 GPMC_D15   IO
AD1   | 87 GPMC_NCS1   O
AE5   | 88 GPMC_D4   IO
B5   | 89 GPMC_NCS6   O
AA2   | 90 GPMC_D0   IO
AD6   | 91 GPMC_D5   IO
AD10   | 92 GPMC_NADV_ALE   O
U2   | 93 GPMC_D11   IO
AA1   | 94 GPMC_D1   IO
B4   | 95 GPMC_NCS4   O
C6   | 96 GPMC_WAIT3   I
N2   | 97 GPMC_NOE   O
AC5   | 98 GPMC_D7   IO
H1   | 99 GPMC_A2   O
AC1   | 100 GPMC_D3   IO
Y1   | 101 GPMC_D9   IO
L2   | 102 GPMC_D14   IO
G2   | 103 GPMC_A4   O
AD8   | 104 GPMC_NCS0   O
E1   | 105 GPMC_A7   O
AC11   | 106 GPMC_WAIT0   I
M1   | 107 GPMC_NWE   O
U1   | 108 GPMC_D12   IO
J1   | 109 GPMC_NBE1   O
A3   | 110 GPMC_NCS2   O
J2   | 111 GPMC_A1   O
F1   | 112 GPMC_A5   O
C5   | 113 GPMC_NCS7   O
T1   | 114 GPMC_D10   IO
N1   | 115 GPMC_CLK   O
AC2   | 116 GPMC_D2   IO
J23   | 117 HDQ_SIO   IO
W20   | 118 HSUSB0_DATA3   IO
V19   | 119 HSUSB0_DIR   I
V20   | 120 HSUSB0_DATA0   IO
V18   | 121 HSUSB0_DATA2   IO
Y18   | 122 HSUSB0_DATA5   IO
U20   | 123 HSUSB0_STP   O
W18   | 124 HSUSB0_NXT   I
Y20   | 125 HSUSB0_DATA1   IO
W17   | 126 HSUSB0_DATA4   IO
Y17   | 127 HSUSB0_DATA7   IO
W19   | 128 HSUSB0_CLK   I
Y19   | 129 HSUSB0_DATA6   IO
W16   | 130 I2C4_SDA   IO
AC4   | 131 I2C3_SDA   IO
C2   | 132 I2C2_SCL   IO
AD15   | 133 I2C4_SCL   IO
J24   | 134 I2C1_SDA   IO
C1   | 135 I2C2_SDA   IO
J25   | 136 I2C1_SCL   IO
AB4   | 137 I2C3_SCL   IO
Y15   | 138 JTAG_EMU0   IO
U16   | 139 JTAG_TDI   I
U15   | 140 JTAG_NTRST   I
V14   | 141 JTAG_TCK   I
V15   | 142 JTAG_TMS_TMSC   IO
Y13   | 143 JTAG_TDO   O
W13   | 144 JTAG_RTCK   O
Y14   | 145 JTAG_EMU1   IO
T19   | 146 MCBSP_CLKS   I
V17   | 147 MCBSP1_FSR   IO
P20   | 148 MCBSP1_FSX   IO
T17   | 149 MCBSP1_CLKX   IO
U19   | 150 MCBSP1_CLKR   IO
U17   | 151 MCBSP1_DX   IO
T20   | 152 MCBSP1_DR   I
R18   | 153 MCBSP2_CLKX   IO
U18   | 154 MCBSP2_FSX   IO
T18   | 155 MCBSP2_DR   I
R19   | 156 MCBSP2_DX   IO
W3   | 157 MCBSP3_FSX   IO
U3   | 158 MCBSP3_CLKX   IO
P3   | 159 MCBSP3_DX   IO
N3   | 160 MCBSP3_DR   I
U4   | 161 MCBSP4_DR   I
V3   | 162 MCBSP4_CLKX   IO
R3   | 163 MCBSP4_DX   IO
T3   | 164 MCBSP4_FSX   IO
R9   | 165 MCSPI1_CS2   O
T8   | 166 MCSPI1_CS3   O
P8   | 167 MCSPI1_SIMO   IO
R8   | 168 MCSPI1_CS1   O
P7   | 169 MCSPI1_SOMI   IO
P9   | 170 MCSPI1_CLK   IO
R7   | 171 MCSPI1_CS0   IO
W7   | 172 MCSPI2_CLK   IO
V9   | 173 MCSPI2_CS1   O
V8   | 174 MCSPI2_CS0   IO
U8   | 175 MCSPI2_SOMI   IO
W8   | 176 MCSPI2_SIMO   IO
L18   | 177 MMC1_CMD   IO
K18   | 178 MMC1_DAT2   IO
N19   | 179 MMC1_CLK   O
M19   | 180 MMC1_DAT0   IO
M18   | 181 MMC1_DAT1   IO
N20   | 182 MMC1_DAT3   IO
V10   | 183 MMC2_DAT4   IO
T9   | 184 MMC2_DAT1   IO
R10   | 185 MMC2_CMD   IO
T10   | 186 MMC2_DAT0   IO
L3   | 187 MMC2_DAT6   IO
U9   | 188 MMC2_DAT3   IO
W10   | 189 MMC2_CLK   O
U10   | 190 MMC2_DAT2   IO
K3   | 191 MMC2_DAT7   IO
M3   | 192 MMC2_DAT5   IO
P18   | 193 gpio_128   O
P19   | 194 gpio_129   O
M20   | 195 gpio_126   IO
P17   | 196 gpio_127   O
W15   | 197 SYS_CLKREQ   IO
E3   | 198 SYS_BOOT3   I
D3   | 199 SYS_BOOT1   I
G3   | 200 SYS_BOOT5   I
AE20   | 201 SYS_32K   I
V16   | 202 SYS_NIRQ   I
V13   | 203 SYS_NRESPWRON   I
AD7   | 204 SYS_NRESWARM   IO
AF19   | 205 SYS_XTALIN   I
AE14   | 206 SYS_CLKOUT1   O
C3   | 207 SYS_BOOT2   I
D4   | 208 SYS_BOOT6   I
E4   | 209 SYS_BOOT4   I
F3   | 210 SYS_BOOT0   I
V12   | 211 SYS_OFF_MODE   O
W11   | 212 SYS_CLKOUT2   O
R2   | 213 UART1_RTS   O
H3   | 214 UART1_RX   I
L4   | 215 UART1_TX   O
W2   | 216 UART1_CTS   I
AA24   | 217 UART2_RTS   O
Y24   | 218 UART2_CTS   I
AD22   | 219 UART2_TX   O
AD21   | 220 UART2_RX   I
H24   | 221 UART3_RX_IRRX   I
G24   | 222 UART3_TX_IRTX   O
F23   | 223 UART3_CTS_RCTX   IO
F24   | 224 UART3_RTS_SD   O
[Model Data]
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[End Model Data]
[End Package Model]
| Models and submodels in the file (271): Model1 (Input), Model2 (I/O), Model3 (I/O), Model4 (I/O), Model5 (I/O), Model6 (I/O), Model7 (I/O), Model8 (I/O), Model9 (I/O), Model10 (I/O), Model11 (Input), Model12 (Input), Model13 (Input), Model14 (I/O), Model15 (I/O), Model16 (I/O), Model17 (I/O), Model18 (I/O), Model19 (I/O), Model20 (I/O), Model21 (I/O), Model22 (I/O), Model23 (I/O), Model24 (I/O), Model25 (I/O), Model26 (I/O), Model27 (I/O), Model28 (I/O), Model29 (I/O), Model30 (I/O), Model31 (I/O), Model32 (I/O), Model33 (I/O), Model34 (I/O), Model35 (I/O), Model36 (I/O), Model37 (I/O), Model38 (I/O), Model39 (I/O), Model40 (I/O), Model41 (I/O), Model42 (I/O), Model43 (I/O), Model44 (I/O), Model45 (I/O), Model46 (I/O), Model47 (I/O), Model48 (I/O), Model49 (I/O), Model50 (I/O), Model51 (I/O), Model52 (I/O), Model53 (I/O), Model54 (I/O), Model55 (I/O), Model56 (I/O), Model57 (I/O), Model58 (I/O), Model59 (I/O), Model60 (I/O), Model61 (I/O), Model62 (I/O), Model63 (I/O), Model64 (I/O), Model65 (I/O), Model66 (I/O), Model67 (I/O), Model68 (I/O), Model69 (I/O), Model70 (I/O), Model71 (I/O), Model72 (I/O), Model73 (I/O), Model74 (I/O), Model75 (I/O), Model76 (I/O), Model77 (I/O), Model78 (I/O), Model79 (I/O), Model80 (I/O)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
